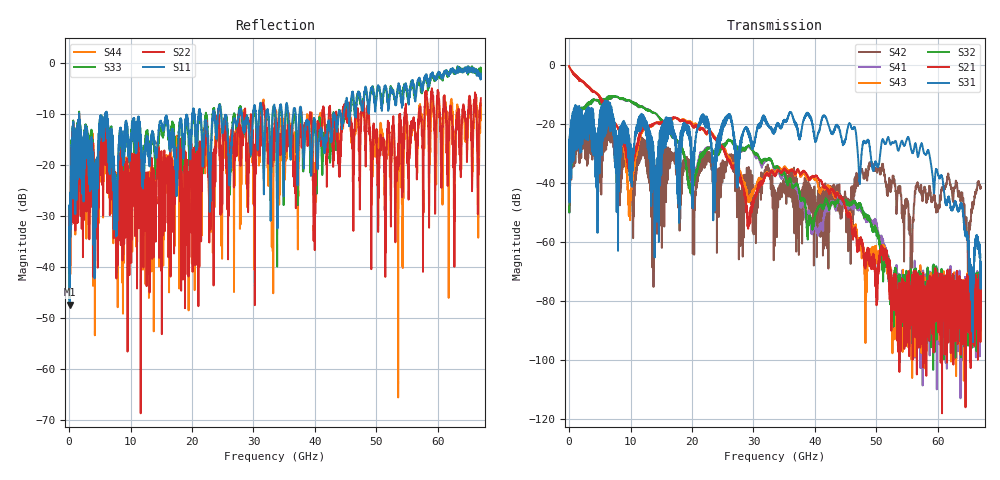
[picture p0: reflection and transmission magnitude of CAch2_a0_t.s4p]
!Agilent Technologies,N5247A,US51170199,A.09.90.13
!Agilent N5247A: A.09.90.13
!Date: Tuesday, October 23, 2018 14:10:07
!Correction: S11(Full 4 Port(1,2,3,4))
!S12(Full 4 Port(1,2,3,4))
!S13(Full 4 Port(1,2,3,4))
!S14(Full 4 Port(1,2,3,4))
!S21(Full 4 Port(1,2,3,4))
!S22(Full 4 Port(1,2,3,4))
!S23(Full 4 Port(1,2,3,4))
!S24(Full 4 Port(1,2,3,4))
!S31(Full 4 Port(1,2,3,4))
!S32(Full 4 Port(1,2,3,4))
!S33(Full 4 Port(1,2,3,4))
!S34(Full 4 Port(1,2,3,4))
!S41(Full 4 Port(1,2,3,4))
!S42(Full 4 Port(1,2,3,4))
!S43(Full 4 Port(1,2,3,4))
!S44(Full 4 Port(1,2,3,4))
!S4P File: Measurements: <S11,S12,S13,S14>,
!<S21,S22,S23,S24>,
!<S31,S32,S33,S34>,
!<S41,S42,S43,S44>:
# Hz S  dB  R 50
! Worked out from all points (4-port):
!   6701 points, 10 MHz to 67 GHz, reference 50 ohm
!   strongest paths, dB at 10 MHz, 16.76 GHz, 33.51 GHz, 50.25 GHz, 67 GHz:
!     S31: -33.3, -23.1, -21.4, -34.5, -70.9
!     S21: -0.4, -17.8, -37.0, -70.7, -73.5
!     S32: -48.3, -23.9, -34.8, -57.7, -79.1
!     S43: -0.3, -18.1, -36.5, -64.2, -82.7
!     S41: -48.5, -24.0, -35.8, -56.8, -81.5
!     S42: -33.5, -31.4, -44.3, -35.5, -41.7
!   lowest |S11| = -47.3 dB at 89.99 MHz (marker M1), VSWR 1.01, Z = 49.9 - j0.424 ohm
!   |S11| at or under -10 dB: 1.641 GHz to 5.89 GHz (4.249 GHz wide, 113 % of centre); 6.102 GHz to 20.05 GHz (13.95 GHz wide, 107 % of centre); 37.85 GHz to 43.09 GHz (5.246 GHz wide, 13 % of centre)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
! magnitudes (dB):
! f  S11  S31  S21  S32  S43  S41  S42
! 10 MHz  -28.3  -33.3  -0.4  -48.3  -0.3  -48.5  -33.5
! 89.99 MHz  -47.3  -33.2  -0.8  -43.4  -0.8  -43.3  -33.5
! 7.669 GHz  -27.7  -25.5  -20.3  -10.6  -20.3  -10.7  -28.2
! 9.839 GHz  -17.8  -32.1  -35.9  -12.0  -50.1  -12.0  -31.7
! 40.24 GHz  -16.7  -25.4  -37.5  -49.6  -38.8  -56.1  -49.5
! 55.12 GHz  -6.8  -24.4  -85.7  -71.1  -74.7  -78.3  -47.3
! 67 GHz  -2.1  -70.9  -73.5  -79.1  -82.7  -81.5  -41.7
